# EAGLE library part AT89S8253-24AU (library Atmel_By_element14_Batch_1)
8-bit Flash Microcontroller
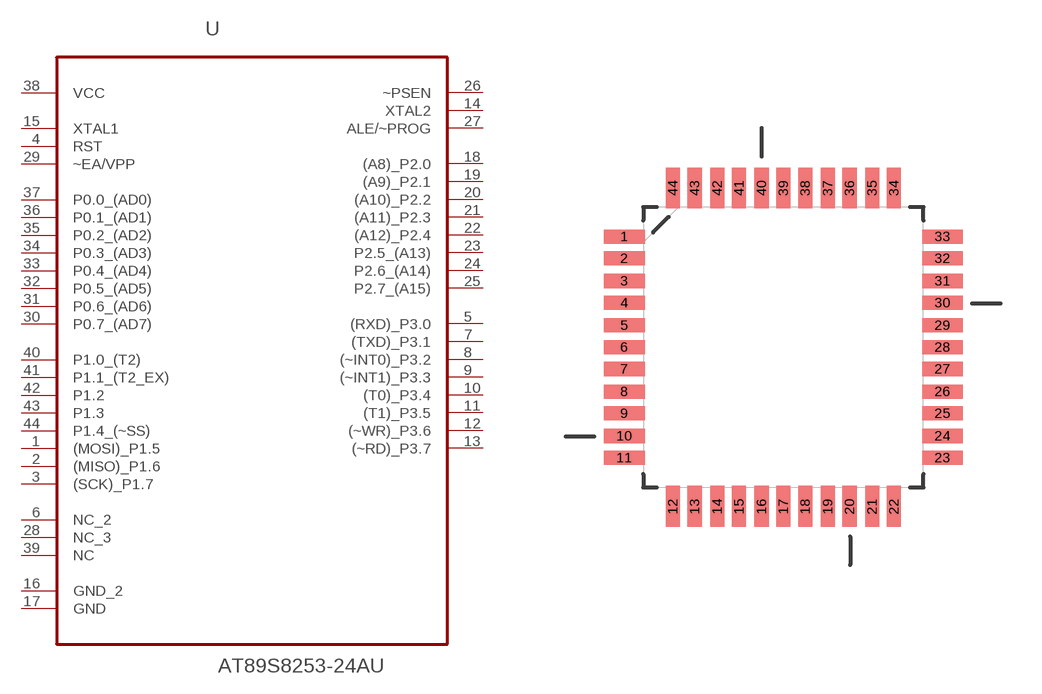
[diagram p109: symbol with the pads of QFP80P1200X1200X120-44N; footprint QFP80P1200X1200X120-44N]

Designator prefix U

## AT89S8253-24AU (DESCRIPTION: 8-bit Flash Microcontroller; MPN: AT89S8253-24AU; OC_FARNELL: 1095744; OC_NEWARK: 74K4052; PACKAGE: VQFP-44; SUPPLIER: ATMEL)  [QFP80P1200X1200X120-44N]
1  (MOSI)_P1.5
2  (MISO)_P1.6
3  (SCK)_P1.7
4  RST  in
5  (RXD)_P3.0
6  NC_2  nc
7  (TXD)_P3.1
8  (~INT0)_P3.2
9  (~INT1)_P3.3
10  (T0)_P3.4
11  (T1)_P3.5
12  (~WR)_P3.6
13  (~RD)_P3.7
14  XTAL2  out
15  XTAL1  in
16  GND_2  pas
17  GND  pas
18  (A8)_P2.0
19  (A9)_P2.1
20  (A10)_P2.2
21  (A11)_P2.3
22  (A12)_P2.4
23  P2.5_(A13)
24  P2.6_(A14)
25  P2.7_(A15)
26  ~PSEN  out
27  ALE/~PROG  out
28  NC_3  nc
29  ~EA/VPP  in
30  P0.7_(AD7)
31  P0.6_(AD6)
32  P0.5_(AD5)
33  P0.4_(AD4)
34  P0.3_(AD3)
35  P0.2_(AD2)
36  P0.1_(AD1)
37  P0.0_(AD0)
38  VCC  pwr
39  NC  nc
40  P1.0_(T2)
41  P1.1_(T2_EX)
42  P1.2
43  P1.3
44  P1.4_(~SS)

## Footprint QFP80P1200X1200X120-44N (pad centres in mm)
smd 1.473 x 0.508: 1 -5.74,3.988; 2 -5.74,3.2; 3 -5.74,2.388; 4 -5.74,1.6; 5 -5.74,0.787; 6 -5.74,0; 7 -5.74,-0.787; 8 -5.74,-1.6; 9 -5.74,-2.388; 10 -5.74,-3.2; 11 -5.74,-3.988; 23 5.74,-3.988; 24 5.74,-3.2; 25 5.74,-2.388; 26 5.74,-1.6; 27 5.74,-0.787; 28 5.74,0; 29 5.74,0.787; 30 5.74,1.6; 31 5.74,2.388; 32 5.74,3.2; 33 5.74,3.988
smd 0.508 x 1.473: 12 -3.988,-5.74; 13 -3.2,-5.74; 14 -2.388,-5.74; 15 -1.6,-5.74; 16 -0.787,-5.74; 17 0,-5.74; 18 0.787,-5.74; 19 1.6,-5.74; 20 2.388,-5.74; 21 3.2,-5.74; 22 3.988,-5.74; 34 3.988,5.74; 35 3.2,5.74; 36 2.388,5.74; 37 1.6,5.74; 38 0.787,5.74; 39 0,5.74; 40 -0.787,5.74; 41 -1.6,5.74; 42 -2.388,5.74; 43 -3.2,5.74; 44 -3.988,5.74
